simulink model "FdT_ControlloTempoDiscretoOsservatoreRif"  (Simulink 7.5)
settings: Solver=FixedStepDiscrete  StartTime=0.0  StopTime=10.0  FixedStep=Ts  RelTol=1e-3
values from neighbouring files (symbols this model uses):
  as1 = 25    [TSC130625ProvaMatlab.m]
  as2 = 10    [TSC130625ProvaMatlab.m]
  Den = [1 -4.427 3.843 -0.2122]    [TSC130625ProvaMatlab.m]
  Kff = -inv(Cz*inv(Az-Bz*K-eye(m))*Bz)    [TSC130625ProvaMatlab.m]
  L = -acker(Az',Cz',[0 0 0])'    [TSC130625ProvaMatlab.m]
  Num = [-0.04181 -0.1416 -0.02034]    [TSC130625ProvaMatlab.m]
  Ts = 0.5    [TSC130625ProvaMatlab.m]
  ts1 = 2    [TSC130625ProvaMatlab.m]
  ts2 = 16    [TSC130625ProvaMatlab.m]
undefined symbols (not defined in the file or in its folder): Az, Bz, Cz, K
libraries: simulink x1

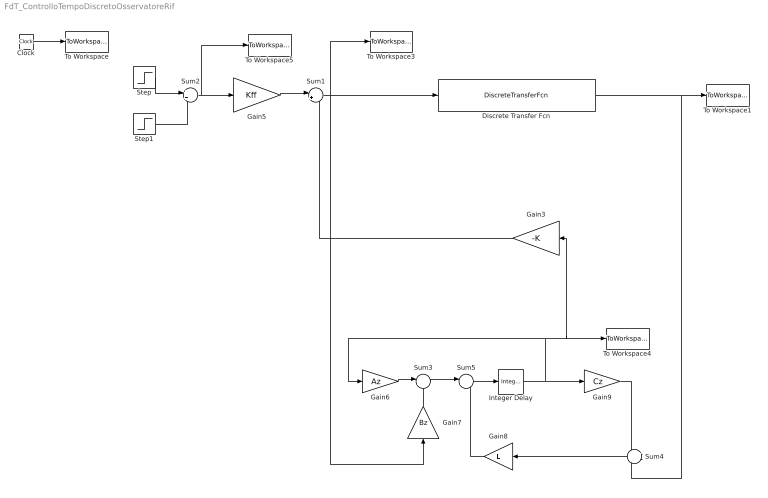
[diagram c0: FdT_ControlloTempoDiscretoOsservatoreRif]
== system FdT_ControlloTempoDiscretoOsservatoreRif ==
  Clock : Clock
  Discrete Transfer Fcn : DiscreteTransferFcn  Numerator=Num  Denominator=Den  SampleTime=Ts
  Gain3 : Gain  Gain=-K  Multiplication=Matrix(K*u)  ParameterDataType=sfix(16)  ParameterScaling=2^0  OutDataType=sfix(16)  OutScaling=2^0
  Gain5 : Gain  Gain=Kff  Multiplication=Matrix(K*u)  ParameterDataType=sfix(16)  ParameterScaling=2^0  OutDataType=sfix(16)  OutScaling=2^0
  Gain6 : Gain  Gain=Az  Multiplication=Matrix(K*u)  ParameterDataType=sfix(16)  ParameterScaling=2^0  OutDataType=sfix(16)  OutScaling=2^0
  Gain7 : Gain  Gain=Bz  Multiplication=Matrix(K*u)  ParameterDataType=sfix(16)  ParameterScaling=2^0  OutDataType=sfix(16)  OutScaling=2^0
  Gain8 : Gain  Gain=L  Multiplication=Matrix(K*u)  ParameterDataType=sfix(16)  ParameterScaling=2^0  OutDataType=sfix(16)  OutScaling=2^0
  Gain9 : Gain  Gain=Cz  Multiplication=Matrix(K*u)  ParameterDataType=sfix(16)  ParameterScaling=2^0  OutDataType=sfix(16)  OutScaling=2^0
  Integer Delay : simulink/Discrete/Integer Delay  vinit=[0 0 0]'  samptime=Ts  NumDelays=1
  Step : Step  Time=ts1  After=as1  SampleTime=0
  Step1 : Step  Time=ts2  After=as2  SampleTime=0
  Sum1 : Sum  Inputs=|++  OutDataType=sfix(16)  OutScaling=2^0
  Sum2 : Sum  OutDataType=sfix(16)  OutScaling=2^0
  Sum3 : Sum  Inputs=|++  OutDataType=sfix(16)  OutScaling=2^0
  Sum4 : Sum  Inputs=+-  OutDataType=sfix(16)  OutScaling=2^0
  Sum5 : Sum  Inputs=|++  OutDataType=sfix(16)  OutScaling=2^0
  To Workspace : ToWorkspace  VariableName=time  SampleTime=-1  SaveFormat=Array
  To Workspace1 : ToWorkspace  VariableName=y  SampleTime=-1  SaveFormat=Array
  To Workspace3 : ToWorkspace  VariableName=ud  SampleTime=-1  SaveFormat=Array
  To Workspace4 : ToWorkspace  VariableName=Xs  SampleTime=-1  SaveFormat=Array
  To Workspace5 : ToWorkspace  VariableName=yref  SampleTime=-1  SaveFormat=Array
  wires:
  Discrete Transfer Fcn/1 -> To Workspace1/1, Sum4/2
  Clock/1 -> To Workspace/1
  Gain6/1 -> Sum3/1
  Integer Delay/1 -> Gain9/1, Gain6/1, Gain3/1, To Workspace4/1
  Gain7/1 -> Sum3/2
  Sum4/1 -> Gain8/1
  Gain9/1 -> Sum4/1
  Gain8/1 -> Sum5/2
  Sum3/1 -> Sum5/1
  Sum5/1 -> Integer Delay/1
  Step/1 -> Sum2/1
  Step1/1 -> Sum2/2
  Sum2/1 -> To Workspace5/1, Gain5/1
  Gain5/1 -> Sum1/1
  Sum1/1 -> Gain7/1, To Workspace3/1, Discrete Transfer Fcn/1
  Gain3/1 -> Sum1/2
